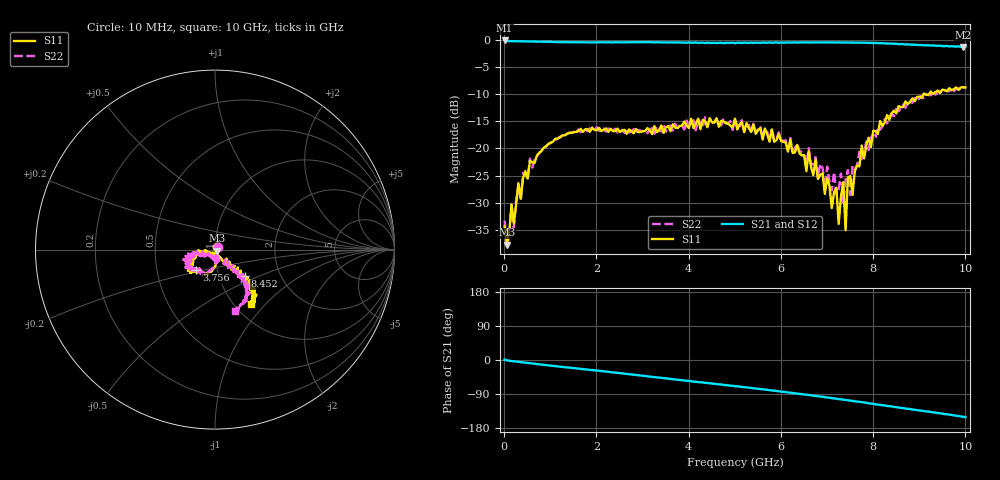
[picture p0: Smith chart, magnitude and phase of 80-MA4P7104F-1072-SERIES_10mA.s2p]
!Agilent Technologies,E8364C,MY48140145,A.09.42.15
!Agilent E8364C: A.09.42.15
!Date: Wednesday, December 02, 2020 07:34:01
!Correction: S11(Full 2 Port(1,2))
!S21(Full 2 Port(1,2))
!S12(Full 2 Port(1,2))
!S22(Full 2 Port(1,2))
!S2P File: Measurements: S11, S21, S12, S22:
# Hz S  dB  R 50
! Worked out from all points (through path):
!   201 points, 10 MHz to 10 GHz, reference 50 ohm
!   highest |S21| = -0.08 dB at 10 MHz (marker M1); lowest = -1.3 dB at 9.95 GHz (marker M2)
!   group delay of S21, straight-line fit = 41 ps
!   lowest |S11| = -37.7 dB at 59.95 MHz (marker M3), VSWR 1.03, Z = 51.2 - j0.621 ohm
!   |S11| at or under -10 dB: start of sweep to 9.092 GHz; 9.13 GHz to 9.209 GHz (78.91 MHz wide, 0.861 % of centre)
!   |S22| runs from -38.0 to -8.7 dB; largest |S21 - S12| = 0.023
!   S11 on the Smith chart (normalised r, x): 10 MHz: 1.03, +0.03; 3.756 GHz: 0.79, -0.18; 8.452 GHz: 1.33, -0.41; 10 GHz: 1.19, -0.83
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1e7  -34.38 44.9  -0.08 1.0  -0.09 -0.3  -33.33 36.1
5.995e7  -37.72 -27.8  -0.19 -1.0  -0.18 -1.0  -38.01 -36.8
1.5985e8  -30.28 -63.4  -0.20 -2.7  -0.20 -2.8  -30.45 -61.8
2.098e8  -33.87 -48.8  -0.21 -3.4  -0.20 -3.5  -34.57 -55.7
3.097e8  -26.39 -76.1  -0.23 -5.0  -0.23 -5.0  -26.70 -73.5
5.5945e8  -22.29 -86.6  -0.28 -8.6  -0.27 -8.7  -21.87 -86.4
1.7083e9  -16.94 -111.5  -0.41 -24.1  -0.39 -23.9  -16.73 -117.2
3.35665e9  -16.68 -131.8  -0.39 -46.3  -0.42 -46.5  -16.71 -125.7
3.75625e9  -16.24 -132.7  -0.43 -52.0  -0.47 -52.1  -16.14 -130.3
5.005e9  -14.52 -149.5  -0.59 -69.1  -0.54 -69.0  -14.63 -162.5
6.7033e9  -24.91 -168.3  -0.42 -94.2  -0.39 -93.9  -22.90 -172.7
7.2028e9  -27.26 -94.7  -0.45 -102.0  -0.42 -101.9  -28.44 -100.0
7.25275e9  -33.89 -129.5  -0.43 -103.2  -0.43 -102.9  -27.49 -138.3
7.35265e9  -26.19 -70.2  -0.47 -104.7  -0.42 -104.4  -30.08 -80.0
7.4026e9  -35.09 -96.3  -0.45 -105.6  -0.45 -105.6  -25.76 -104.6
7.45255e9  -25.35 -78.2  -0.46 -106.0  -0.46 -106.4  -24.00 -70.0
7.5025e9  -25.10 -55.6  -0.46 -107.4  -0.44 -107.0  -28.59 -69.1
7.7023e9  -23.30 -56.7  -0.48 -110.4  -0.50 -110.8  -20.58 -58.8
8.35165e9  -14.71 -39.5  -0.63 -121.9  -0.66 -121.9  -14.01 -50.2
8.45155e9  -13.03 -41.5  -0.69 -123.9  -0.65 -123.3  -14.02 -47.0
9.95005e9  -8.71 -53.4  -1.26 -150.0  -1.27 -149.7  -8.65 -72.1
1e10  -8.75 -56.2  -1.25 -150.8  -1.24 -150.8  -8.84 -71.8
